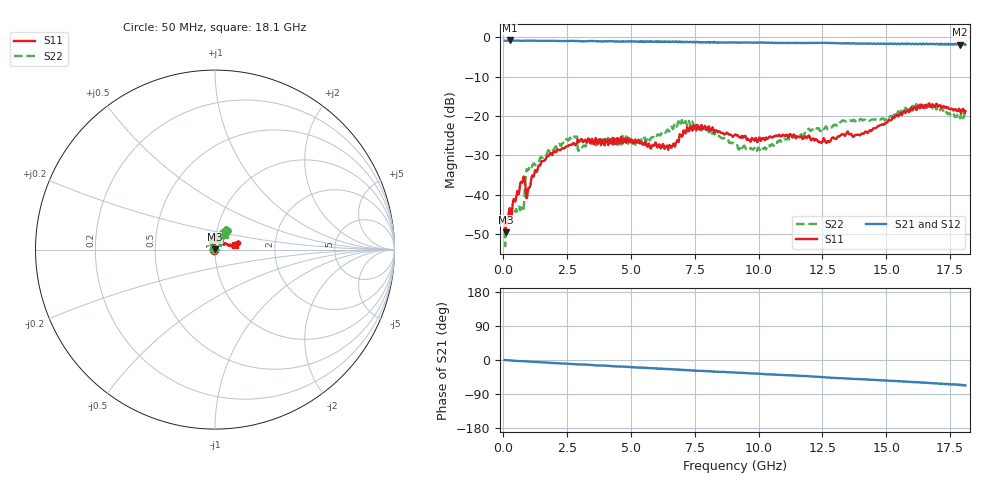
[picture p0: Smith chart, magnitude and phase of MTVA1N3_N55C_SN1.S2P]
! Network Analyzer HP8720D.06.14 Serial No. US36140669
! 10 Jan 2005  15:03:03
! Frequency  S11  S21  S12  S22
# HZ  S  DB R 50
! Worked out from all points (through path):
!   801 points, 50 MHz to 18.1 GHz, reference 50 ohm
!   highest |S21| = -0.86 dB at 253.1 MHz (marker M1); lowest = -2.0 dB at 17.9 GHz (marker M2)
!   group delay of S21, straight-line fit = 9.95 ps
!   lowest |S11| = -49.5 dB at 95.12 MHz (marker M3), VSWR 1.01, Z = 49.7 + j0.199 ohm
!   |S11| at or under -10 dB: start of sweep to end of sweep
!   |S22| runs from -53.0 to -16.9 dB; largest |S21 - S12| = 0.023
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5e7  -47.12 -152.2  -0.91 -0.0  -0.90 -0.5  -45.62 157.0
9.5125e7  -49.50 143.4  -0.93 -0.5  -0.90 -0.9  -48.52 157.6
2.530625e8  -43.34 127.5  -0.86 -0.9  -0.85 -1.3  -44.96 145.5
7.26875e8  -36.94 94.4  -0.95 -3.0  -0.93 -3.4  -42.75 133.8
9.299375e8  -40.59 91.0  -0.90 -3.6  -0.92 -4.0  -33.58 142.6
9.97625e8  -38.11 95.6  -0.91 -4.1  -0.90 -4.4  -33.40 135.3
1.178125e9  -35.38 104.0  -0.90 -5.1  -0.93 -5.4  -32.03 124.0
1.76475e9  -30.19 93.1  -0.91 -7.0  -0.93 -7.3  -28.68 113.7
2.802625e9  -27.34 81.3  -1.02 -11.1  -0.99 -11.6  -25.42 110.7
3.073375e9  -25.90 83.2  -1.01 -11.9  -0.98 -12.2  -27.89 121.3
6.074188e9  -27.73 95.6  -1.17 -23.3  -1.16 -23.1  -24.66 108.4
6.63825e9  -27.25 104.7  -1.16 -25.0  -1.19 -24.8  -23.32 96.0
7.202312e9  -22.78 99.8  -1.17 -27.0  -1.21 -27.0  -22.46 70.5
7.834062e9  -23.27 92.9  -1.31 -28.6  -1.25 -29.4  -23.02 54.2
9.075e9  -24.73 111.6  -1.40 -32.9  -1.35 -33.2  -27.25 41.2
9.954938e9  -26.62 107.4  -1.39 -35.7  -1.37 -36.4  -28.39 41.4
1.209838e10  -25.96 73.0  -1.46 -43.4  -1.44 -43.8  -23.39 69.5
1.403875e10  -24.48 34.0  -1.67 -50.8  -1.64 -51.2  -20.96 70.1
1.509919e10  -20.91 16.8  -1.70 -55.1  -1.59 -54.8  -20.43 72.1
1.640781e10  -17.21 12.1  -1.84 -58.7  -1.65 -59.3  -17.81 59.4
1.789694e10  -18.45 12.2  -1.95 -65.0  -1.99 -65.4  -20.60 60.9
1.81e10  -18.75 14.2  -1.92 -67.3  -1.89 -68.3  -20.23 55.0
